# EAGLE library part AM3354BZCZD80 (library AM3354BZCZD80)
Sitara processor: Arm Cortex-A8, 3D graphics, CAN Source: Datasheet
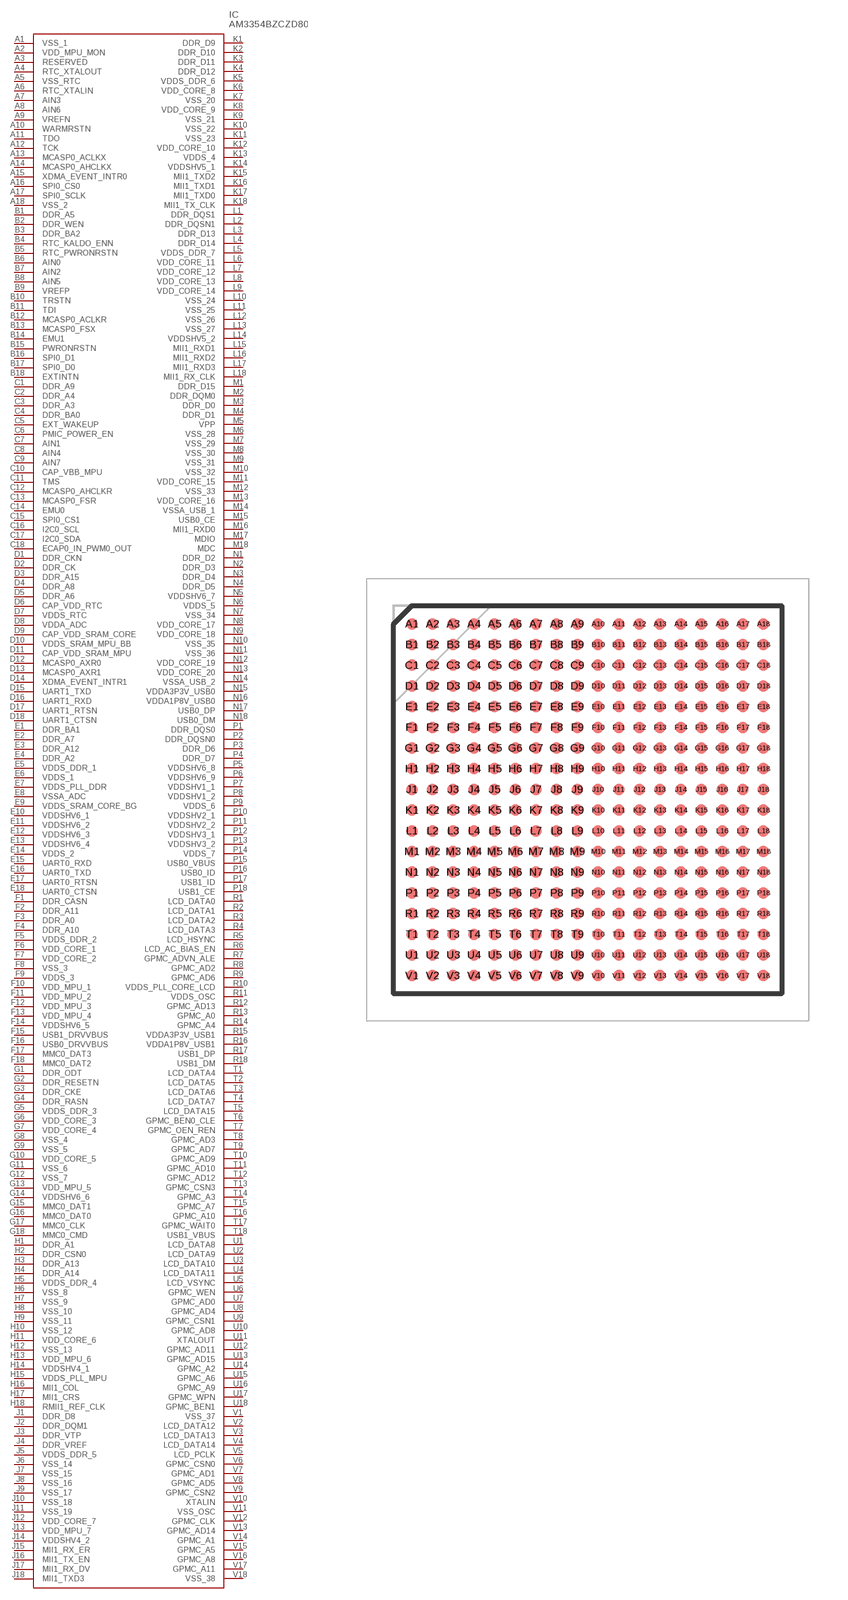
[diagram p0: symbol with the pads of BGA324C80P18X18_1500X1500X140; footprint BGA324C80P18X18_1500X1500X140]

Designator prefix IC

## AM3354BZCZD80 (Description: <p>Sitara processor: Arm Cortex-A8, 3D graphics, CAN</p>; Height: 1.4mm; Manufacturer_Name: Texas Instruments; Manufacturer_Part_Number: AM3354BZCZD80; Mouser_Part_Number: 595-AM3354BZCZD80; Mouser_Price-Stock: https://www.mouser.co.uk/ProductDetail/Texas-Instruments/AM3354BZCZD80?qs=OHhYoCux73kJgJV%252ByKiEdQ%3D%3D)  [BGA324C80P18X18_1500X1500X140]
A1  VSS_1
A2  VDD_MPU_MON
A3  RESERVED
A4  RTC_XTALOUT
A5  VSS_RTC
A6  RTC_XTALIN
A7  AIN3
A8  AIN6
A9  VREFN
A10  WARMRSTN
A11  TDO
A12  TCK
A13  MCASP0_ACLKX
A14  MCASP0_AHCLKX
A15  XDMA_EVENT_INTR0
A16  SPI0_CS0
A17  SPI0_SCLK
A18  VSS_2
B1  DDR_A5
B2  DDR_WEN
B3  DDR_BA2
B4  RTC_KALDO_ENN
B5  RTC_PWRONRSTN
B6  AIN0
B7  AIN2
B8  AIN5
B9  VREFP
B10  TRSTN
B11  TDI
B12  MCASP0_ACLKR
B13  MCASP0_FSX
B14  EMU1
B15  PWRONRSTN
B16  SPI0_D1
B17  SPI0_D0
B18  EXTINTN
C1  DDR_A9
C2  DDR_A4
C3  DDR_A3
C4  DDR_BA0
C5  EXT_WAKEUP
C6  PMIC_POWER_EN
C7  AIN1
C8  AIN4
C9  AIN7
C10  CAP_VBB_MPU
C11  TMS
C12  MCASP0_AHCLKR
C13  MCASP0_FSR
C14  EMU0
C15  SPI0_CS1
C16  I2C0_SCL
C17  I2C0_SDA
C18  ECAP0_IN_PWM0_OUT
D1  DDR_CKN
D2  DDR_CK
D3  DDR_A15
D4  DDR_A8
D5  DDR_A6
D6  CAP_VDD_RTC
D7  VDDS_RTC
D8  VDDA_ADC
D9  CAP_VDD_SRAM_CORE
D10  VDDS_SRAM_MPU_BB
D11  CAP_VDD_SRAM_MPU
D12  MCASP0_AXR0
D13  MCASP0_AXR1
D14  XDMA_EVENT_INTR1
D15  UART1_TXD
D16  UART1_RXD
D17  UART1_RTSN
D18  UART1_CTSN
E1  DDR_BA1
E2  DDR_A7
E3  DDR_A12
E4  DDR_A2
E5  VDDS_DDR_1
E6  VDDS_1
E7  VDDS_PLL_DDR
E8  VSSA_ADC
E9  VDDS_SRAM_CORE_BG
E10  VDDSHV6_1
E11  VDDSHV6_2
E12  VDDSHV6_3
E13  VDDSHV6_4
E14  VDDS_2
E15  UART0_RXD
E16  UART0_TXD
E17  UART0_RTSN
E18  UART0_CTSN
F1  DDR_CASN
F2  DDR_A11
F3  DDR_A0
F4  DDR_A10
F5  VDDS_DDR_2
F6  VDD_CORE_1
F7  VDD_CORE_2
F8  VSS_3
F9  VDDS_3
F10  VDD_MPU_1
F11  VDD_MPU_2
F12  VDD_MPU_3
F13  VDD_MPU_4
F14  VDDSHV6_5
F15  USB1_DRVVBUS
F16  USB0_DRVVBUS
F17  MMC0_DAT3
F18  MMC0_DAT2
G1  DDR_ODT
G2  DDR_RESETN
G3  DDR_CKE
G4  DDR_RASN
G5  VDDS_DDR_3
G6  VDD_CORE_3
G7  VDD_CORE_4
G8  VSS_4
G9  VSS_5
G10  VDD_CORE_5
G11  VSS_6
G12  VSS_7
G13  VDD_MPU_5
G14  VDDSHV6_6
G15  MMC0_DAT1
G16  MMC0_DAT0
G17  MMC0_CLK
G18  MMC0_CMD
H1  DDR_A1
H2  DDR_CSN0
H3  DDR_A13
H4  DDR_A14
H5  VDDS_DDR_4
H6  VSS_8
H7  VSS_9
H8  VSS_10
H9  VSS_11
H10  VSS_12
H11  VDD_CORE_6
H12  VSS_13
H13  VDD_MPU_6
H14  VDDSHV4_1
H15  VDDS_PLL_MPU
H16  MII1_COL
H17  MII1_CRS
H18  RMII1_REF_CLK
J1  DDR_D8
J2  DDR_DQM1
J3  DDR_VTP
J4  DDR_VREF
J5  VDDS_DDR_5
J6  VSS_14
J7  VSS_15
J8  VSS_16
J9  VSS_17
J10  VSS_18
J11  VSS_19
J12  VDD_CORE_7
J13  VDD_MPU_7
J14  VDDSHV4_2
J15  MII1_RX_ER
J16  MII1_TX_EN
J17  MII1_RX_DV
J18  MII1_TXD3
K1  DDR_D9
K2  DDR_D10
K3  DDR_D11
K4  DDR_D12
K5  VDDS_DDR_6
K6  VDD_CORE_8
K7  VSS_20
K8  VDD_CORE_9
K9  VSS_21
K10  VSS_22
K11  VSS_23
K12  VDD_CORE_10
K13  VDDS_4
K14  VDDSHV5_1
K15  MII1_TXD2
K16  MII1_TXD1
K17  MII1_TXD0
K18  MII1_TX_CLK
L1  DDR_DQS1
L2  DDR_DQSN1
L3  DDR_D13
L4  DDR_D14
L5  VDDS_DDR_7
L6  VDD_CORE_11
L7  VDD_CORE_12
L8  VDD_CORE_13
L9  VDD_CORE_14
L10  VSS_24
L11  VSS_25
L12  VSS_26
L13  VSS_27
L14  VDDSHV5_2
L15  MII1_RXD1
L16  MII1_RXD2
L17  MII1_RXD3
L18  MII1_RX_CLK
M1  DDR_D15
M2  DDR_DQM0
M3  DDR_D0
M4  DDR_D1
M5  VPP
M6  VSS_28
M7  VSS_29
M8  VSS_30
M9  VSS_31
M10  VSS_32
M11  VDD_CORE_15
M12  VSS_33
M13  VDD_CORE_16
M14  VSSA_USB_1
M15  USB0_CE
M16  MII1_RXD0
M17  MDIO
M18  MDC
N1  DDR_D2
N2  DDR_D3
N3  DDR_D4
N4  DDR_D5
N5  VDDSHV6_7
N6  VDDS_5
N7  VSS_34
N8  VDD_CORE_17
N9  VDD_CORE_18
N10  VSS_35
N11  VSS_36
N12  VDD_CORE_19
N13  VDD_CORE_20
N14  VSSA_USB_2
N15  VDDA3P3V_USB0
N16  VDDA1P8V_USB0
N17  USB0_DP
N18  USB0_DM
P1  DDR_DQS0
P2  DDR_DQSN0
P3  DDR_D6
P4  DDR_D7
P5  VDDSHV6_8
P6  VDDSHV6_9
P7  VDDSHV1_1
P8  VDDSHV1_2
P9  VDDS_6
P10  VDDSHV2_1
P11  VDDSHV2_2
P12  VDDSHV3_1
P13  VDDSHV3_2
P14  VDDS_7
P15  USB0_VBUS
P16  USB0_ID
P17  USB1_ID
P18  USB1_CE
R1  LCD_DATA0
R2  LCD_DATA1
R3  LCD_DATA2
R4  LCD_DATA3
R5  LCD_HSYNC
R6  LCD_AC_BIAS_EN
R7  GPMC_ADVN_ALE
R8  GPMC_AD2
R9  GPMC_AD6
R10  VDDS_PLL_CORE_LCD
R11  VDDS_OSC
R12  GPMC_AD13
R13  GPMC_A0
R14  GPMC_A4
R15  VDDA3P3V_USB1
R16  VDDA1P8V_USB1
R17  USB1_DP
R18  USB1_DM
T1  LCD_DATA4
T2  LCD_DATA5
T3  LCD_DATA6
T4  LCD_DATA7
T5  LCD_DATA15
T6  GPMC_BEN0_CLE
T7  GPMC_OEN_REN
T8  GPMC_AD3
T9  GPMC_AD7
T10  GPMC_AD9
T11  GPMC_AD10
T12  GPMC_AD12
T13  GPMC_CSN3
T14  GPMC_A3
T15  GPMC_A7
T16  GPMC_A10
T17  GPMC_WAIT0
T18  USB1_VBUS
U1  LCD_DATA8
U2  LCD_DATA9
U3  LCD_DATA10
U4  LCD_DATA11
U5  LCD_VSYNC
U6  GPMC_WEN
U7  GPMC_AD0
U8  GPMC_AD4
U9  GPMC_CSN1
U10  GPMC_AD8
U11  XTALOUT
U12  GPMC_AD11
U13  GPMC_AD15
U14  GPMC_A2
U15  GPMC_A6
U16  GPMC_A9
U17  GPMC_WPN
U18  GPMC_BEN1
V1  VSS_37
V2  LCD_DATA12
V3  LCD_DATA13
V4  LCD_DATA14
V5  LCD_PCLK
V6  GPMC_CSN0
V7  GPMC_AD1
V8  GPMC_AD5
V9  GPMC_CSN2
V10  XTALIN
V11  VSS_OSC
V12  GPMC_CLK
V13  GPMC_AD14
V14  GPMC_A1
V15  GPMC_A5
V16  GPMC_A8
V17  GPMC_A11
V18  VSS_38

## Footprint BGA324C80P18X18_1500X1500X140 (pad centres in mm)
ZCZ (S-PBGA-N324)
smd 0.45 x 0.45: A1 -6.8,6.8; A2 -6,6.8; A3 -5.2,6.8; A4 -4.4,6.8; A5 -3.6,6.8; A6 -2.8,6.8; A7 -2,6.8; A8 -1.2,6.8; A9 -0.4,6.8; A10 0.4,6.8; A11 1.2,6.8; A12 2,6.8; A13 2.8,6.8; A14 3.6,6.8; A15 4.4,6.8; A16 5.2,6.8; A17 6,6.8; A18 6.8,6.8; B1 -6.8,6; B2 -6,6; B3 -5.2,6; B4 -4.4,6; B5 -3.6,6; B6 -2.8,6; B7 -2,6; B8 -1.2,6; B9 -0.4,6; B10 0.4,6; B11 1.2,6; B12 2,6; B13 2.8,6; B14 3.6,6; B15 4.4,6; B16 5.2,6; B17 6,6; B18 6.8,6; C1 -6.8,5.2; C2 -6,5.2; C3 -5.2,5.2; C4 -4.4,5.2; C5 -3.6,5.2; C6 -2.8,5.2; C7 -2,5.2; C8 -1.2,5.2; C9 -0.4,5.2; C10 0.4,5.2; C11 1.2,5.2; C12 2,5.2; C13 2.8,5.2; C14 3.6,5.2; C15 4.4,5.2; C16 5.2,5.2; C17 6,5.2; C18 6.8,5.2; D1 -6.8,4.4; D2 -6,4.4; D3 -5.2,4.4; D4 -4.4,4.4; D5 -3.6,4.4; D6 -2.8,4.4; D7 -2,4.4; D8 -1.2,4.4; D9 -0.4,4.4; D10 0.4,4.4; D11 1.2,4.4; D12 2,4.4; D13 2.8,4.4; D14 3.6,4.4; D15 4.4,4.4; D16 5.2,4.4; D17 6,4.4; D18 6.8,4.4; E1 -6.8,3.6; E2 -6,3.6; E3 -5.2,3.6; E4 -4.4,3.6; E5 -3.6,3.6; E6 -2.8,3.6; E7 -2,3.6; E8 -1.2,3.6; E9 -0.4,3.6; E10 0.4,3.6; E11 1.2,3.6; E12 2,3.6; E13 2.8,3.6; E14 3.6,3.6; E15 4.4,3.6; E16 5.2,3.6; E17 6,3.6; E18 6.8,3.6; F1 -6.8,2.8; F2 -6,2.8; F3 -5.2,2.8; F4 -4.4,2.8; F5 -3.6,2.8; F6 -2.8,2.8; F7 -2,2.8; F8 -1.2,2.8; F9 -0.4,2.8; F10 0.4,2.8; F11 1.2,2.8; F12 2,2.8; F13 2.8,2.8; F14 3.6,2.8; F15 4.4,2.8; F16 5.2,2.8; F17 6,2.8; F18 6.8,2.8; G1 -6.8,2; G2 -6,2; G3 -5.2,2; G4 -4.4,2; G5 -3.6,2; G6 -2.8,2; G7 -2,2; G8 -1.2,2; G9 -0.4,2; G10 0.4,2; G11 1.2,2; G12 2,2; G13 2.8,2; G14 3.6,2; G15 4.4,2; G16 5.2,2; G17 6,2; G18 6.8,2; H1 -6.8,1.2; H2 -6,1.2; H3 -5.2,1.2; H4 -4.4,1.2; H5 -3.6,1.2; H6 -2.8,1.2; H7 -2,1.2; H8 -1.2,1.2; H9 -0.4,1.2; H10 0.4,1.2; H11 1.2,1.2; H12 2,1.2; H13 2.8,1.2; H14 3.6,1.2; H15 4.4,1.2; H16 5.2,1.2; H17 6,1.2; H18 6.8,1.2; J1 -6.8,0.4; J2 -6,0.4; J3 -5.2,0.4; J4 -4.4,0.4; J5 -3.6,0.4; J6 -2.8,0.4; J7 -2,0.4; J8 -1.2,0.4; J9 -0.4,0.4; J10 0.4,0.4; J11 1.2,0.4; J12 2,0.4; J13 2.8,0.4; J14 3.6,0.4; J15 4.4,0.4; J16 5.2,0.4; J17 6,0.4; J18 6.8,0.4; K1 -6.8,-0.4; K2 -6,-0.4; K3 -5.2,-0.4; K4 -4.4,-0.4; K5 -3.6,-0.4; K6 -2.8,-0.4; K7 -2,-0.4; K8 -1.2,-0.4; K9 -0.4,-0.4; K10 0.4,-0.4; K11 1.2,-0.4; K12 2,-0.4; K13 2.8,-0.4; K14 3.6,-0.4; K15 4.4,-0.4; K16 5.2,-0.4; K17 6,-0.4; K18 6.8,-0.4; L1 -6.8,-1.2; L2 -6,-1.2; L3 -5.2,-1.2; L4 -4.4,-1.2; L5 -3.6,-1.2; L6 -2.8,-1.2; L7 -2,-1.2; L8 -1.2,-1.2; L9 -0.4,-1.2; L10 0.4,-1.2; L11 1.2,-1.2; L12 2,-1.2; L13 2.8,-1.2; L14 3.6,-1.2; L15 4.4,-1.2; L16 5.2,-1.2; L17 6,-1.2; L18 6.8,-1.2; M1 -6.8,-2; M2 -6,-2; M3 -5.2,-2; M4 -4.4,-2; M5 -3.6,-2; M6 -2.8,-2; M7 -2,-2; M8 -1.2,-2; M9 -0.4,-2; M10 0.4,-2; M11 1.2,-2; M12 2,-2; M13 2.8,-2; M14 3.6,-2; M15 4.4,-2; M16 5.2,-2; M17 6,-2; M18 6.8,-2; N1 -6.8,-2.8; N2 -6,-2.8; N3 -5.2,-2.8; N4 -4.4,-2.8; N5 -3.6,-2.8; N6 -2.8,-2.8; N7 -2,-2.8; N8 -1.2,-2.8; N9 -0.4,-2.8; N10 0.4,-2.8; N11 1.2,-2.8; N12 2,-2.8; N13 2.8,-2.8; N14 3.6,-2.8; N15 4.4,-2.8; N16 5.2,-2.8; N17 6,-2.8; N18 6.8,-2.8; P1 -6.8,-3.6; P2 -6,-3.6; P3 -5.2,-3.6; P4 -4.4,-3.6; P5 -3.6,-3.6; P6 -2.8,-3.6; P7 -2,-3.6; P8 -1.2,-3.6; P9 -0.4,-3.6; P10 0.4,-3.6; P11 1.2,-3.6; P12 2,-3.6; P13 2.8,-3.6; P14 3.6,-3.6; P15 4.4,-3.6; P16 5.2,-3.6; P17 6,-3.6; P18 6.8,-3.6; R1 -6.8,-4.4; R2 -6,-4.4; R3 -5.2,-4.4; R4 -4.4,-4.4; R5 -3.6,-4.4; R6 -2.8,-4.4; R7 -2,-4.4; R8 -1.2,-4.4; R9 -0.4,-4.4; R10 0.4,-4.4; R11 1.2,-4.4; R12 2,-4.4; R13 2.8,-4.4; R14 3.6,-4.4; R15 4.4,-4.4; R16 5.2,-4.4; R17 6,-4.4; R18 6.8,-4.4; T1 -6.8,-5.2; T2 -6,-5.2; T3 -5.2,-5.2; T4 -4.4,-5.2; T5 -3.6,-5.2; T6 -2.8,-5.2; T7 -2,-5.2; T8 -1.2,-5.2; T9 -0.4,-5.2; T10 0.4,-5.2; T11 1.2,-5.2; T12 2,-5.2; T13 2.8,-5.2; T14 3.6,-5.2; T15 4.4,-5.2; T16 5.2,-5.2; T17 6,-5.2; T18 6.8,-5.2; U1 -6.8,-6; U2 -6,-6; U3 -5.2,-6; U4 -4.4,-6; U5 -3.6,-6; U6 -2.8,-6; U7 -2,-6; U8 -1.2,-6; U9 -0.4,-6; U10 0.4,-6; U11 1.2,-6; U12 2,-6; U13 2.8,-6; U14 3.6,-6; U15 4.4,-6; U16 5.2,-6; U17 6,-6; U18 6.8,-6; V1 -6.8,-6.8; V2 -6,-6.8; V3 -5.2,-6.8; V4 -4.4,-6.8; V5 -3.6,-6.8; V6 -2.8,-6.8; V7 -2,-6.8; V8 -1.2,-6.8; V9 -0.4,-6.8; V10 0.4,-6.8; V11 1.2,-6.8; V12 2,-6.8; V13 2.8,-6.8; V14 3.6,-6.8; V15 4.4,-6.8; V16 5.2,-6.8; V17 6,-6.8; V18 6.8,-6.8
